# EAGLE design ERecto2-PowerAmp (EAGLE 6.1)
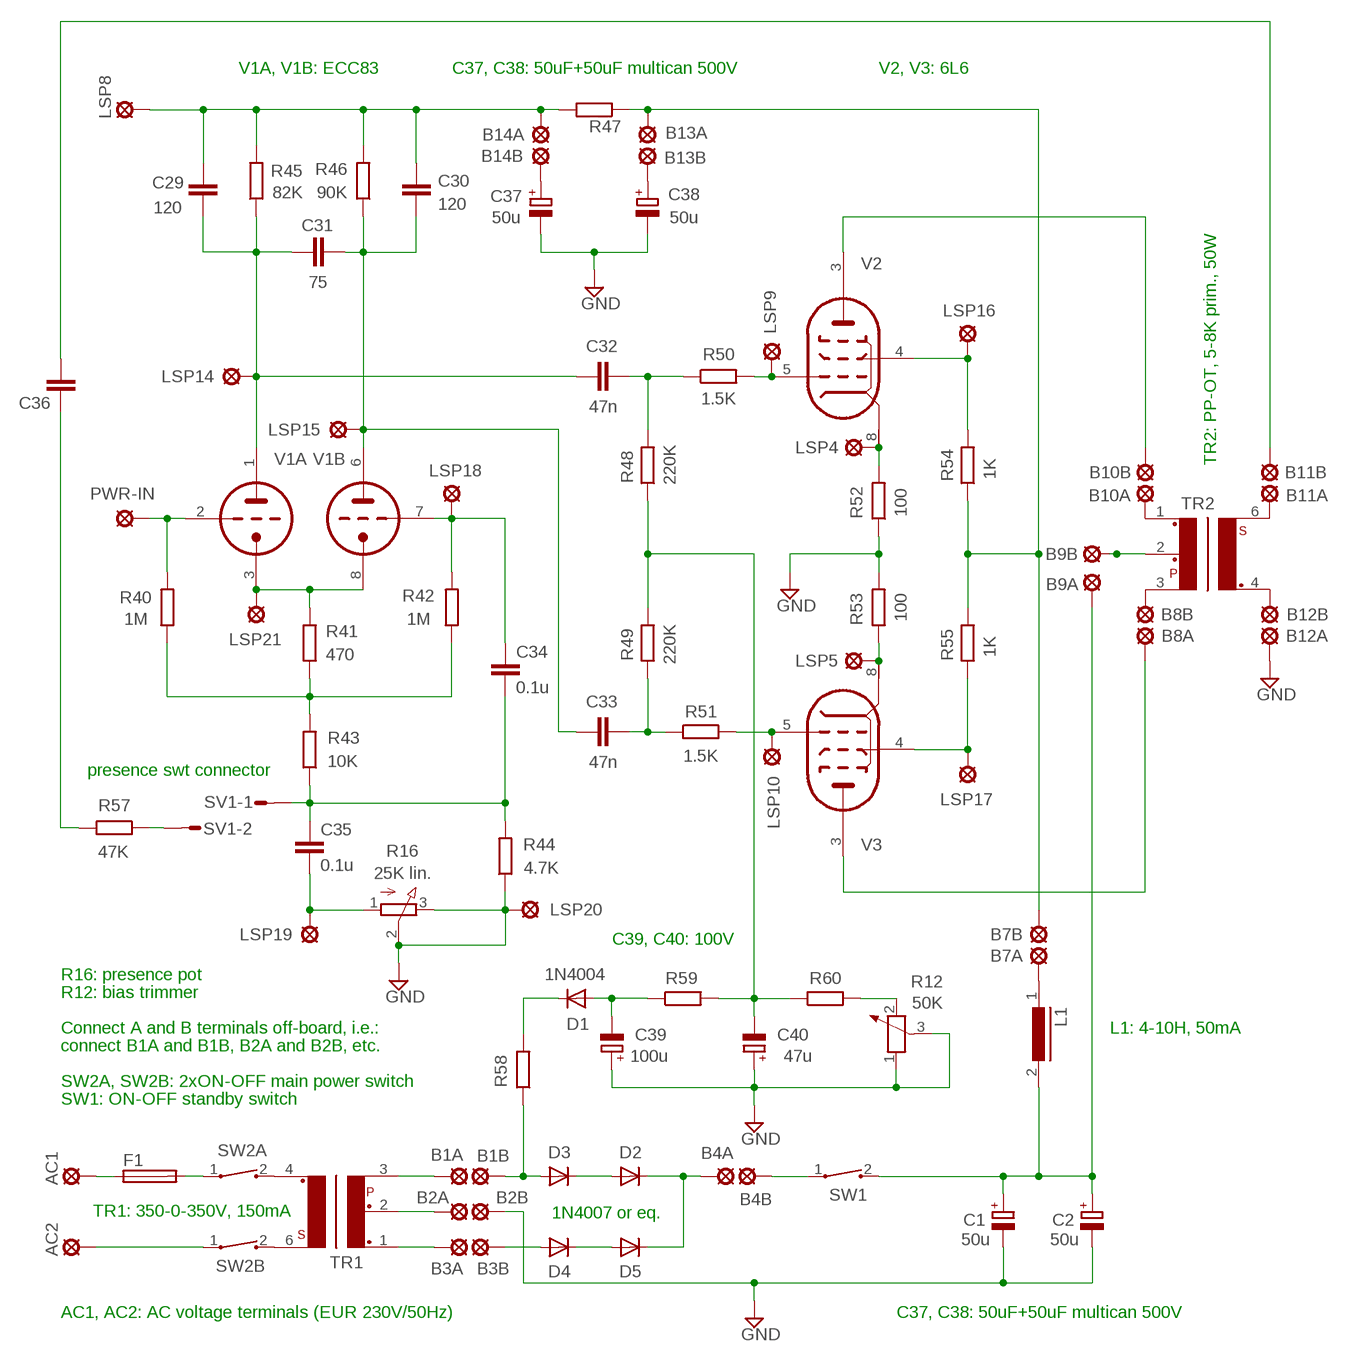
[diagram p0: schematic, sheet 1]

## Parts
AC1  LSP13  [LSP13]
AC2  LSP13  [LSP13]
B1A  LSP13  [LSP13]
B1B  LSP13  [LSP13]
B2A  LSP13  [LSP13]
B2B  LSP13  [LSP13]
B3A  LSP13  [LSP13]
B3B  LSP13  [LSP13]
B4A  LSP13  [LSP13]
B4B  LSP13  [LSP13]
B7A  LSP13  [LSP13]
B7B  LSP13  [LSP13]
B8A  LSP13  [LSP13]
B8B  LSP13  [LSP13]
B9A  LSP13  [LSP13]
B9B  LSP13  [LSP13]
B10A  LSP13  [LSP13]
B10B  LSP13  [LSP13]
B11A  LSP13  [LSP13]
B11B  LSP13  [LSP13]
B12A  LSP13  [LSP13]
B12B  LSP13  [LSP13]
B13A  LSP13  [LSP13]
B13B  LSP13  [LSP13]
B14A  LSP13  [LSP13]
B14B  LSP13  [LSP13]
C1  50u  CPOL-EUE10-35  [EB35D]
C2  50u  CPOL-EUE10-35  [EB35D]
C29  120  C-EU102-054X133  [C102-054X133]
C30  120  C-EU102-054X133  [C102-054X133]
C31  75  C-EU102-054X133  [C102-054X133]
C32  47n  C22/7  [C22.5B7]
C33  47n  C22/7  [C22.5B7]
C34  0.1u  C-EU102-054X133  [C102-054X133]
C35  0.1u  C-EU102-054X133  [C102-054X133]
C36  C-EU102-054X133  [C102-054X133]
C37  50u  CPOL-EUE5-8.5  [E5-8,5]
C38  50u  CPOL-EUE5-8.5  [E5-8,5]
C39  100u  CPOL-EUE5-8.5  [E5-8,5]
C40  47u  CPOL-EUE5-8.5  [E5-8,5]
D1  1N4004  [DO41-10]
D2  1N4004  [DO41-10]
D3  1N4004  [DO41-10]
D4  1N4004  [DO41-10]
D5  1N4004  [DO41-10]
F1  FUSEF456  [F456]
L1  82114A  [82114A]
LSP4  LSP13  [LSP13]
LSP5  LSP13  [LSP13]
LSP8  LSP13  [LSP13]
LSP9  LSP13  [LSP13]
LSP10  LSP13  [LSP13]
LSP14  LSP13  [LSP13]
LSP15  LSP13  [LSP13]
LSP16  LSP13  [LSP13]
LSP17  LSP13  [LSP13]
LSP18  LSP13  [LSP13]
LSP19  LSP13  [LSP13]
LSP20  LSP13  [LSP13]
LSP21  LSP13  [LSP13]
PWR-IN  LSP13  [LSP13]
R12  50K  POTENTIOMETER_PT-10  [PT-10]
R16  25K lin.  3RP/1610N  [3RP/1610N]
R40  1M  R-EU_0207/12  [0207/12]
R41  470  R-EU_0207/10  [0207/10]
R42  1M  R-EU_0207/12  [0207/12]
R43  10K  R-EU_0207/12  [0207/12]
R44  4.7K  R-EU_0207/10  [0207/10]
R45  82K  R-EU_0411/15  [0411/15]
R46  90K  R-EU_0411/15  [0411/15]
R47  R-EU_0617/22  [0617/22]
R48  220K  R-EU_0207/12  [0207/12]
R49  220K  R-EU_0207/12  [0207/12]
R50  1.5K  R-EU_0207/12  [0207/12]
R51  1.5K  R-EU_0207/12  [0207/12]
R52  100  R-EU_0617/17  [0617/17]
R53  100  R-EU_0617/17  [0617/17]
R54  1K  R-EU_0617/22  [0617/22]
R55  1K  R-EU_0617/22  [0617/22]
R57  47K  R-EU_0207/10  [0207/10]
R58  R-EU_0207/12  [0207/12]
R59  R-EU_0207/12  [0207/12]
R60  R-EU_0207/12  [0207/12]
SV1  S02P  [S02P]
SW1  CT10-XXXX-A2  [CT10-XXXX-A2]
SW2A  CT10-XXXX-A2  [CT10-XXXX-A2]
SW2B  CT10-XXXX-A2  [CT10-XXXX-A2]
TR1  42TM113  [42TM]
TR2  42TM113  [42TM]
V1  ECC83-P  [NOVAL]
V2  6L6GC-P  [OKTAL]
V3  6L6GC-P  [OKTAL]

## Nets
GND: B2B.MP B12A.MP C1.- C2.- C37.- C38.- C39.+ C40.+ LSP20.MP R12.1 R12.3 R16.2(S) R16.3(E) R44.1 R52.1 R53.2
N$1: LSP4.MP R52.2 V2.8(PK)
N$2: B4A.MP D2.C D5.C
N$3: LSP5.MP R53.1 V3.8(PK)
N$4: LSP17.MP R55.1 V3.4(PSG)
N$5: LSP16.MP R54.2 V2.4(PSG)
N$6: B14A.MP C29.2 C30.1 LSP8.MP R45.2 R46.2 R47.2
N$7: LSP10.MP R51.2 V3.5(PG)
N$8: LSP9.MP R50.2 V2.5(PG)
N$9: C32.2 R48.2 R50.1
N$10: B10B.MP V2.3(PA)
N$11: C33.2 R49.1 R51.1
N$12: C40.- R48.1 R49.2 R59.2 R60.1
N$13: C39.- D1.A R59.1
N$14: D1.C R58.2
N$15: R12.2 R60.2
N$16: B8A.MP V3.3(PA)
N$17: B7B.MP B13A.MP R47.1 R54.1 R55.2
N$18: D2.A D3.C
N$19: D4.C D5.A
N$20: B1B.MP D3.A R58.1
N$21: B3B.MP D4.A
N$22: C30.2 C31.2 C33.1 LSP15.MP R46.1 V1.6(B:TA)
N$23: C29.1 C31.1 C32.1 LSP14.MP R45.1 V1.1(A:TA)
N$24: LSP21.MP R41.2 V1.3(A:TK) V1.8(B:TK)
N$25: C34.1 LSP18.MP R42.2 V1.7(B:TG)
N$26: R40.1 R41.1 R42.1 R43.2
N$27: C35.2 LSP19.MP R16.1(A)
N$28: C34.2 C35.1 R43.1 R44.2 SV1.1
N$29: R57.1 SV1.2
N$30: C36.1 R57.2
N$31: B11B.MP C36.2
N$32: B9A.MP C1.+ C2.+ L1.2 SW1.2
N$33: B1A.MP TR1.3
N$34: B2A.MP TR1.2
N$35: F1.2 SW2A.1
N$36: AC1.MP F1.1
N$37: AC2.MP SW2B.1
N$38: B3A.MP TR1.1
N$39: PWR-IN.MP R40.2 V1.2(A:TG)
N$40: SW2A.2 TR1.4
N$41: SW2B.2 TR1.6
N$42: B4B.MP SW1.1
N$44: B8B.MP TR2.3
N$45: B9B.MP TR2.2
N$46: B10A.MP TR2.1
N$47: B11A.MP TR2.6
N$48: B12B.MP TR2.4
N$49: B7A.MP L1.1
N$51: B13B.MP C38.+
N$52: B14B.MP C37.+
Unconnected: V1.4(":H1) V1.5(":H3) V1.9(":H2) V2.2(H1) V2.7(H2) V3.2(H1) V3.7(H2)

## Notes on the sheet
- V1A, V1B: ECC83 | C37, C38: 50uF+50uF multican 500V | V2, V3: 6L6
- TR2: PP-OT, 5-8K prim., 50W
- presence swt connector
- C39, C40: 100V
- R16: presence pot
- R12: bias trimmer
- Connect A and B terminals off-board, i.e.: | L1: 4-10H, 50mA
- connect B1A and B1B, B2A and B2B, etc.
- SW2A, SW2B: 2xON-OFF main power switch
- SW1: ON-OFF standby switch
- TR1: 350-0-350V, 150mA | 1N4007 or eq.
- AC1, AC2: AC voltage terminals (EUR 230V/50Hz) | C37, C38: 50uF+50uF multican 500V

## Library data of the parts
AC1 AC2 B1A B1B B2A B2B B3A B3B B4A B4B B7A B7B B8A B8B B9A B9B B10A B10B B11A B11B B12A B12B B13A B13B B14A B14B LSP4 LSP5 LSP8-LSP10 LSP14-LSP21 PWR-IN = solpad:LSP13: SOLDER PAD
C1 C2 C37-C40 = rcl:CPOL-EU: POLARIZED CAPACITOR, European symbol
C29-C31 C34-C36 = rcl:C-EU: CAPACITOR, European symbol
C32 C33 = capacitor-wima:C: CAPACITOR
D1-D5 = diode:1N4004: DIODE
F1 = fuse:FUSE: Fuse; OC_FARNELL: unknown; OC_NEWARK: unknown
L1 = inductors:82114A: INDUCTOR
R12 = rcl:POTENTIOMETER_: Potentiometer
R16 = pot:3RP/1610N: 16mm Potentiometer one level Source: http://www.alphapotentiometers.net/html/16mm_pot_2.html
R40-R55 R57-R60 = rcl:R-EU_: RESISTOR, European symbol
SV1 = con-amp-mt:S02P: AMP MT CONNECTOR; OC_FARNELL: unknown; OC_NEWARK: unknown
SW1 SW2A SW2B = switch-coto:CT10-XXXX-: CT10 Series Molded Switch
TR1 TR2 = trafo-xicon:42TM113: Transformer Mouser 42TLM Series Source: http://www.mouser.com/catalog/specsheets/164267.pdf; OC_FARNELL: unknown; OC_NEWARK: unknown
V1 = tubes:ECC83-P
V2 V3 = tubes:6L6GC-P

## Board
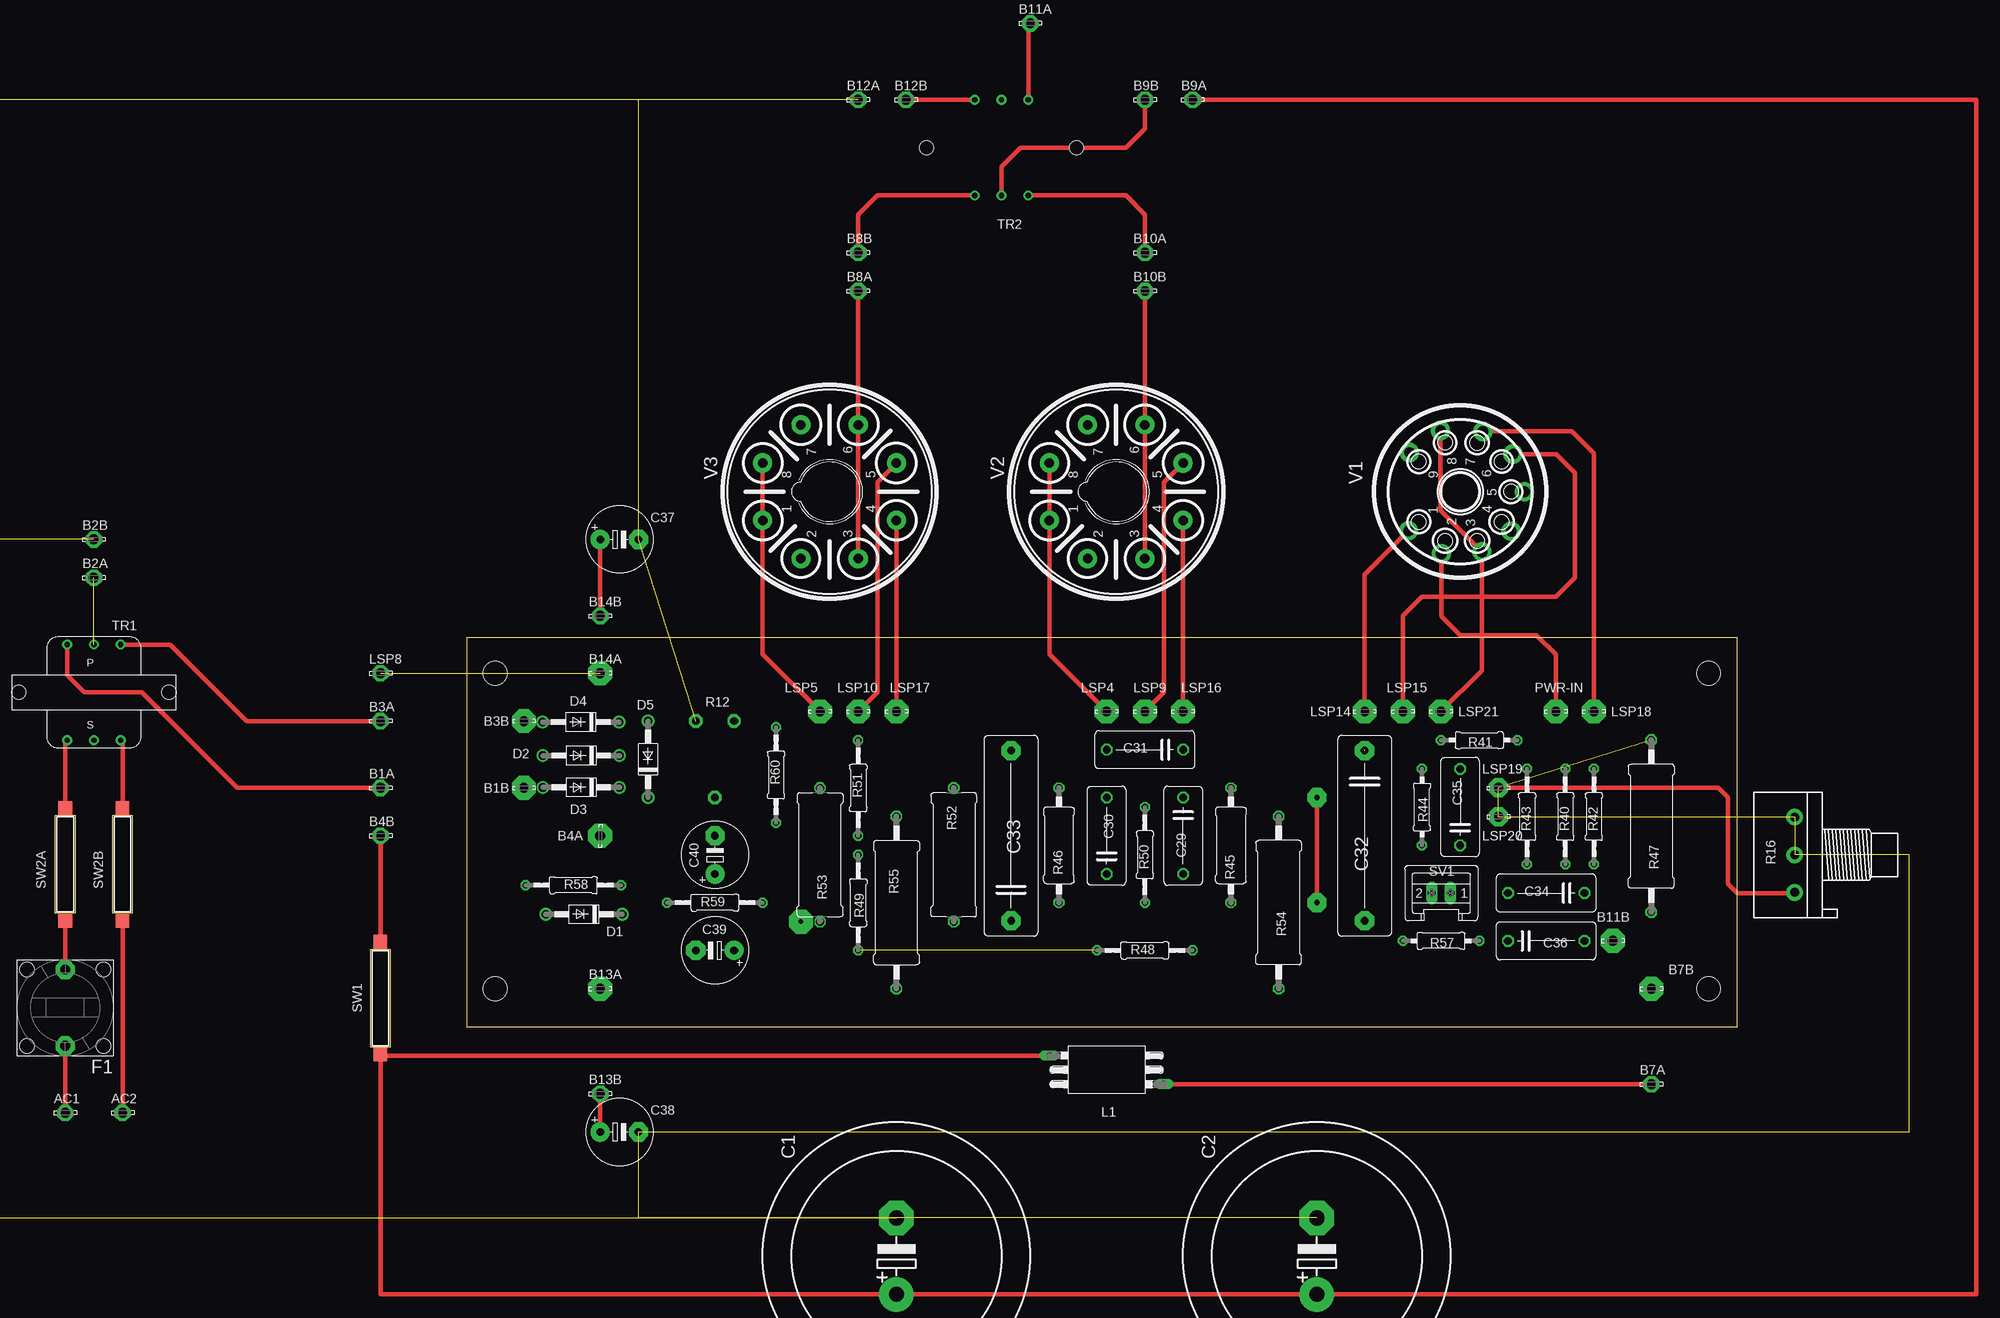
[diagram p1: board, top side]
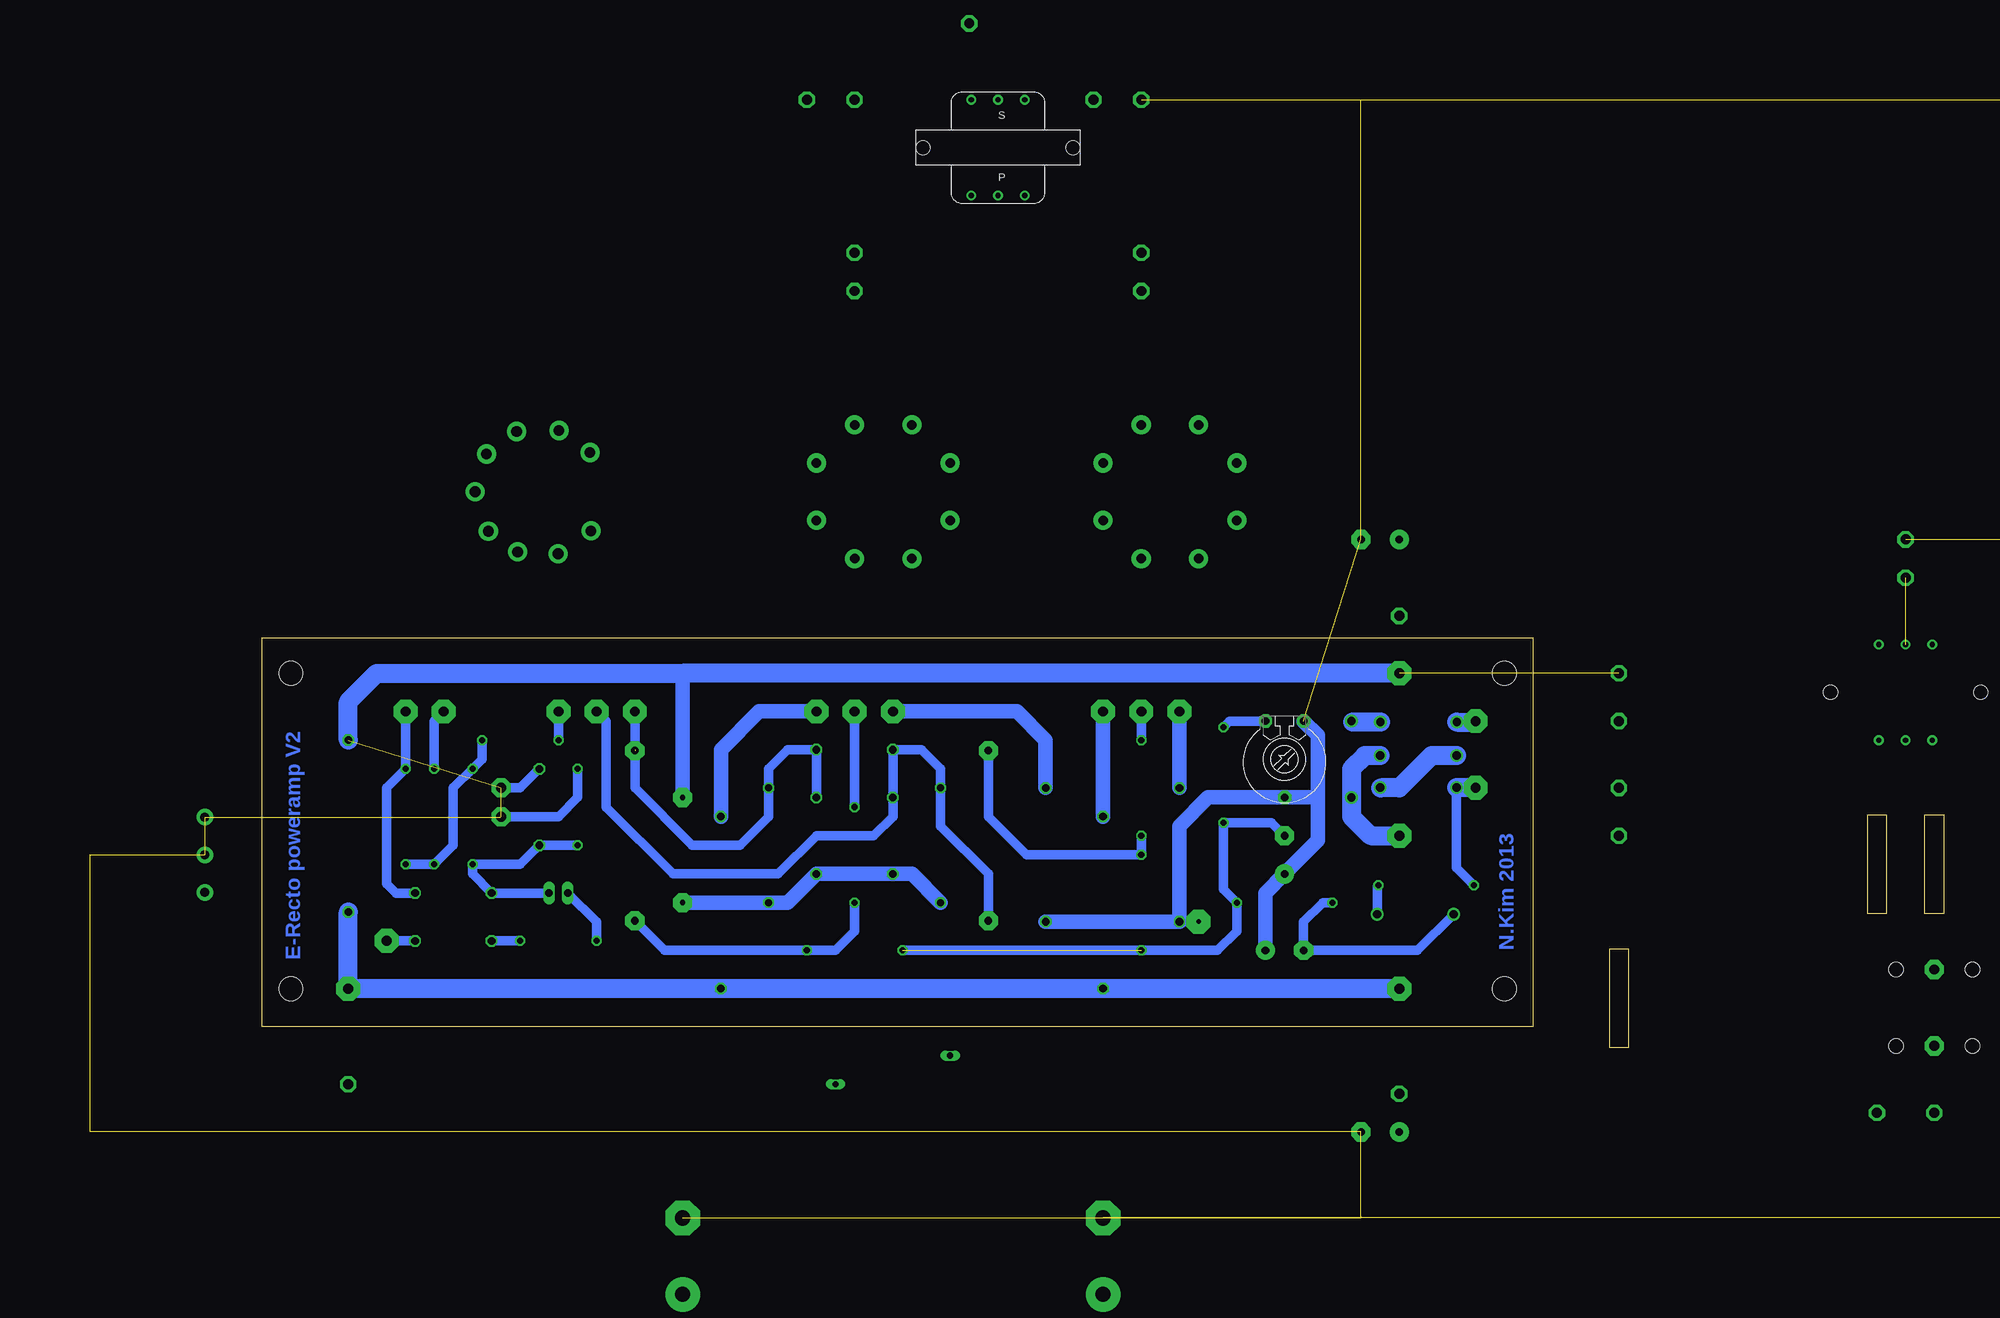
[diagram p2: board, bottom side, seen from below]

Size 223.53 x 54.43 mm. Coordinates in mm from the lower left corner, seen from the top.
Outline: 54.64,2.69 223.53,2.69 223.53,54.43 54.64,54.43 54.64,2.69
Copper layers (1*16): Top 0.035mm / dielectric 1.5mm / Bottom 0.035mm
Design rules: minimum track width 10mil, minimum drill 24mil, track to track 8mil, track to pad 8mil, pad to pad 8mil, via to via 8mil, smd to smd 8mil, copper to edge 40mil, drill to drill 8mil, minimum pad ring 10mil, minimum via ring 8mil, stop-mask expansion 4mil, vias tented up to drill 0mil, thermal gap 10mil
Holes 3.2 mm at 219.74,49.68 219.74,7.77 58.45,49.68 58.45,7.77

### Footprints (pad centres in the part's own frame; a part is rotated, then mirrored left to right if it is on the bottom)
LSP13 = drill 1.321 pad 2.159 octagon: MP 0,0
EB35D = drill 2.007 pad 4.597: + -5.08,0 | drill 2.007 pad 4.597 octagon: - 5.08,0
C102-054X133 = drill 1.016 octagon: 1 -5.08,0; 2 5.08,0
C22.5B7 = drill 1.016 pad 2.54 octagon: 1 -11.303,0; 2 11.303,0
E5-8,5 = drill 1.016 pad 2.54: + -2.54,0 | drill 1.016 pad 2.54 octagon: - 2.54,0
DO41-10 = drill 1.118: A 5.08,0; C -5.08,0
F456 = drill 1.321 pad 2.54 octagon: 1 0,5.08; 2 0,-5.08 | hole 2.007: 5.08,5.08; 5.08,-5.08; -5.08,-5.08; -5.08,5.08
82114A = drill 0.813 long: 1 -7.62,1.905; 2 7.62,-1.905
PT-10 = drill 1.016 pad 1.778 octagon: 1 -2.54,-5.08; 2 2.54,-5.08; 3 0,5.08
3RP/1610N = drill 1.2 pad 2.184: 1 -5,0; 2 0,0; 3 5,0
0207/12 = drill 0.813 octagon: 1 -6.35,0; 2 6.35,0
0207/10 = drill 0.813 octagon: 1 -5.08,0; 2 5.08,0
0411/15 = drill 0.914 octagon: 1 -7.62,0; 2 7.62,0
0617/22 = drill 1.016 octagon: 1 -11.43,0; 2 11.43,0
0617/17 = drill 1.016 octagon: 1 -8.89,0; 2 8.89,0
S02P = drill 1.016 long: 1 1.25,0; 2 -1.25,0
CT10-XXXX-A2 = smd 1.8 x 1.8: 1 -7.5,0; 2 7.5,0
42TM = drill 0.7 pad 1.3: 1 -3.556,-6.35; 2 0,-6.35; 3 3.556,-6.35; 4 3.556,6.35; 5 0,6.35; 6 -3.556,6.35 | hole 1.9: -9.982,0; 9.982,0
NOVAL = drill 1.422 pad 2.54: 1 5.207,-6.858; 2 8.254,-2.484; 3 8.004,2.893; 4 5.258,6.77; 5 0,8.524; 6 -5.004,7.024; 7 -8.004,3.02; 8 -8.127,-2.611; 9 -5.207,-6.731
OKTAL = drill 1.27 pad 2.54: 1 3.81,-8.89; 2 8.89,-3.81; 3 8.89,3.81; 4 3.81,8.89; 5 -3.81,8.89; 6 -8.89,3.81; 7 -8.89,-3.81; 8 -3.81,-8.89

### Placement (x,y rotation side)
AC1  1.3,-8.74 0 top  (outside the outline)
AC2  8.92,-8.74 0 top  (outside the outline)
B1A  43.21,34.44 0 top
B1B  62.26,34.44 0 top
B2A  not placed on the board
B2B  not placed on the board
B3A  43.21,43.33 0 top
B3B  62.26,43.33 0 top
B4A  72.42,28.09 90 top
B4B  43.21,28.09 0 top
B7A  212.12,-4.93 0 top  (outside the outline)
B7B  212.12,7.77 0 top
B8A  106.71,100.48 0 top  (outside the outline)
B8B  106.71,105.56 0 top  (outside the outline)
B9A  151.16,125.88 0 top  (outside the outline)
B9B  144.81,125.88 0 top  (outside the outline)
B10A  144.81,105.56 0 top  (outside the outline)
B10B  144.81,100.48 0 top  (outside the outline)
B11A  129.57,136.04 0 top  (outside the outline)
B11B  207.04,14.12 0 top
B12A  not placed on the board
B12B  113.06,125.88 0 top  (outside the outline)
B13A  72.42,7.77 0 top
B13B  72.42,-6.2 0 top  (outside the outline)
B14A  72.42,49.68 0 top
B14B  72.42,57.3 0 top
C1  111.79,-27.79 90 top  (outside the outline)
C2  167.67,-27.79 90 top  (outside the outline)
C29  149.89,28.09 270 top
C30  139.73,28.09 90 top
C31  144.81,39.52 180 top
C32  174.02,28.09 270 top
C33  127.03,28.09 90 top
C34  198.15,20.47 180 top
C35  186.72,31.9 90 top
C36  198.15,14.12 0 top
C37  74.96,67.46 0 top  (outside the outline)
C38  74.96,-11.28 0 top  (outside the outline)
C39  87.66,12.85 180 top
C40  87.66,25.55 90 top
D1  70.26,17.66 180 top
D2  69.88,38.75 180 top
D3  69.88,34.52 180 top
D4  69.84,43.2 180 top
D5  78.77,38.25 90 top
F1  1.3,5.23 180 top
L1  139.73,-3.02 180 top
LSP4  139.73,44.6 0 top
LSP5  101.63,44.6 0 top
LSP8  43.21,49.68 0 top
LSP9  144.81,44.6 0 top
LSP10  106.71,44.6 0 top
LSP14  174.02,44.6 0 top
LSP15  179.1,44.6 0 top
LSP16  149.89,44.6 0 top
LSP17  111.79,44.6 0 top
LSP18  204.5,44.6 0 top
LSP19  191.8,34.44 0 top
LSP20  191.8,30.63 0 top
LSP21  184.18,44.6 0 top
PWR-IN  199.42,44.6 0 top
R12  87.66,38.25 180 bottom
R16  231.17,25.55 90 top  (outside the outline)
R40  200.69,30.63 90 top
R41  189.26,40.79 180 top
R42  204.5,30.63 90 top
R43  195.61,30.63 90 top
R44  181.64,31.9 270 top
R45  156.24,26.82 270 top
R46  133.38,26.82 270 top
R47  212.12,29.36 90 top
R48  144.81,12.85 0 top
R49  106.71,19.2 270 top
R50  144.81,25.55 90 top
R51  106.71,34.44 90 top
R52  119.41,25.55 90 top
R53  101.63,25.55 270 top
R54  162.59,19.2 90 top
R55  111.79,19.2 270 top
R57  184.18,14.12 0 top
R58  68.85,21.52 0 top
R59  87.66,19.2 0 top
R60  95.78,36.17 90 top
SV1  184.18,20.47 0 top
SW1  43.21,6.5 270 top
SW2A  1.3,24.28 90 top
SW2B  8.92,24.28 90 top
TR1  5.11,47.14 180 top
TR2  125.76,119.53 0 bottom  (outside the outline)
V1  186.72,73.81 270 top  (outside the outline)
V2  141,73.81 270 top  (outside the outline)
V3  102.9,73.81 270 top  (outside the outline)

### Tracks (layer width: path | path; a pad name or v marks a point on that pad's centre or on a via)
GND  (via drill 0.6 pad 3.17)  (16 unrouted)
  Top 0.61: 191.88,30.55 LSP20.MP
  Bottom 1.27: LSP20.MP 184.18,30.63 181.64,33.17 R44.1 | R53.2 v99.09,16.66
  Bottom 1.93: R52.1 R53.2 101.63,29.36 97.82,33.17 R12.3 83.22,33.17 | C39.+ 90.2,20.47 C40.+ 83.22,27.46 83.22,33.17 | 83.22,33.17 83.22,41.43 R12.1
  other vias: 62.26,43.33 62.26,34.44 72.42,49.68 72.42,7.77 101.63,44.6 106.71,44.6 111.79,44.6 174.02,44.6 179.1,44.6 184.18,44.6 139.73,44.6 144.81,44.6 149.89,44.6 199.42,44.6 204.5,44.6 212.12,7.77 207.04,14.12 72.42,28.09
N$1
  Top 0.61: V2.8 132.11,52.22 LSP4.MP
  Bottom 1.93: R52.2 119.41,40.79 123.22,44.6 LSP4.MP
N$2
  Bottom 2.54: D2.C 77,38.75 78.77,36.98 D5.C 78.77,30.63 76.23,28.09 B4A.MP
N$3
  Top 0.61: V3.8 94.01,52.22 LSP5.MP
  Bottom 1.93: R53.1 LSP5.MP
N$4
  Top 0.61: V3.4 LSP17.MP
  Bottom 1.93: LSP17.MP R55.1
N$5
  Top 0.61: V2.4 LSP16.MP
  Bottom 1.93: R54.2 162.59,39.52 157.51,44.6 LSP16.MP
N$6  (via drill 0.7 pad 2.54)  (3 unrouted)
  Top 0.61: v167.67,19.2 v167.67,33.17
  Bottom 1.93: v167.67,33.17 167.67,49.68 | v167.67,19.2 R45.2 153.7,19.2 C29.2 C30.1 137.19,23.01 R46.2
  Bottom 2.54: R47.2 212.12,45.87 208.31,49.68 167.67,49.68 B14A.MP
  other vias: 191.8,34.44 191.8,30.63
N$7
  Top 0.61: V3.5 109.25,75.08 109.25,47.14 LSP10.MP
  Bottom 1.27: R51.2 LSP10.MP
N$8
  Top 0.61: V2.5 147.35,75.08 147.35,47.14 LSP9.MP
  Bottom 1.27: R50.2 LSP9.MP
N$9
  Bottom 1.27: R50.1 144.81,15.39 147.35,12.85 R48.2 170.08,12.85 C32.2
N$10
  Top 0.61: V2.3 B10B.MP
N$11
  Bottom 1.27: R51.1 R49.1 121.95,25.55 127.03,30.63 C33.2
N$12  (1 unrouted)
  Bottom 1.27: C40.- 89.39,29.82 R60.1 95.78,20.97 R59.2 94.01,15.39 96.55,12.85 R48.1
N$13
  Bottom 1.27: R59.1 82.58,19.2 85.12,16.66 C39.- 69.99,12.85 D1.A
N$14
  Bottom 1.27: D1.C 75.34,21.38 R58.2
N$15
  Bottom 1.27: R12.2 94.97,43.33 R60.2
N$16
  Top 0.61: V3.3 B8A.MP
N$17
  Bottom 2.54: R47.1 B7B.MP R54.1 R55.2 B13A.MP
N$18
  Bottom 1.27: 74.88,34.44 D3.C
  Bottom 2.54: D2.A 68.11,38.75 72.42,34.44 74.88,34.44
N$19
  Bottom 1.27: 78.64,43.2 D5.A
  Bottom 2.54: D4.C 78.64,43.2
N$20
  Bottom 1.27: D3.A 64.8,23.82 R58.1
  Bottom 2.54: D3.A 62.34,34.52 B1B.MP
N$21
  Bottom 2.54: D4.A 62.26,43.2 B3B.MP
N$22
  Top 0.61: V1.6 199.5,78.81 201.96,76.35 201.96,62.38 199.42,59.84 181.64,59.84 179.1,57.3 LSP15.MP
  Bottom 1.27: LSP15.MP 177.83,43.33 177.83,31.9 168.94,23.01 154.97,23.01 149.89,28.09 142.27,28.09 139.73,30.63 C30.2 C31.2 135.92,39.52 133.38,36.98 R46.1 133.38,29.36 127.03,23.01 C33.1
N$23  (1 unrouted)
  Top 0.61: V1.1 174.02,62.76 LSP14.MP
  Bottom 1.27: C29.1 C31.1 153.7,39.52 156.24,36.98 R45.1 156.24,30.63 160.05,26.82 166.4,26.82 174.02,34.44 174.02,39.52 LSP14.MP
N$24
  Top 0.61: LSP21.MP 189.61,50.03 V1.3 184.11,71.31 V1.8
  Bottom 1.27: R41.2 LSP21.MP
N$25
  Top 0.61: V1.7 201.58,81.81 204.5,78.89 LSP18.MP
  Bottom 1.27: C34.1 205.77,20.47 207.04,21.74 207.04,34.44 R42.2 LSP18.MP
N$26
  Bottom 1.27: R41.1 194.34,38.25 R43.2 198.15,34.44 198.15,26.82 R40.1 R42.1
N$27
  Top 0.61: LSP19.MP 221.01,34.44 222.28,33.17 222.28,21.74 223.55,20.47 231.09,20.47 R16.1
  Bottom 1.27: LSP19.MP 189.26,34.44 C35.2
N$28
  Bottom 1.27: R44.2 C35.1 189.26,24.28 R43.1 195.61,23.01 C34.2 SV1.1
N$29
  Bottom 1.27: SV1.2 179.1,16.64 R57.1
N$30
  Bottom 1.27: R57.2 C36.1
N$31
  Bottom 1.27: B11B.MP C36.2
N$32
  Top 0.61: B9A.MP 255.3,125.88 255.3,-32.87 C2.+ C1.+ 43.21,-32.87 SW1.2 43.21,-1.12 L1.2
N$33
  Top 0.61: TR1.3 1.55,49.43 3.84,47.14 11.46,47.14 24.16,34.44 B1A.MP
N$34  (1 unrouted)
N$35
  Top 0.61: F1.2 SW2A.1
N$36
  Top 0.61: AC1.MP F1.1
N$37
  Top 0.61: AC2.MP SW2B.1
N$38
  Top 0.61: TR1.1 15.27,53.49 25.43,43.33 B3A.MP
N$39
  Top 0.61: V1.2 184.24,57.24 186.72,54.76 196.88,54.76 199.42,52.22 PWR-IN.MP
  Bottom 1.27: R40.2 200.69,43.33 PWR-IN.MP
N$40
  Top 0.61: SW2A.2 1.3,40.54 TR1.4
N$41
  Top 0.61: SW2B.2 8.92,40.54 TR1.6
N$42
  Top 0.61: SW1.1 B4B.MP
N$44
  Top 0.61: TR2.3 109.25,113.18 106.71,110.64 B8B.MP
N$45
  Top 0.61: TR2.2 125.76,116.99 128.3,119.53 142.27,119.53 144.81,122.07 B9B.MP
N$46
  Top 0.61: TR2.1 142.27,113.18 144.81,110.64 B10A.MP
N$47
  Top 0.61: TR2.6 129.32,136.04 B11A.MP
N$48
  Top 0.61: TR2.4 B12B.MP
N$49
  Top 0.61: L1.1 B7A.MP
N$51
  Top 0.61: C38.+ B13B.MP
N$52
  Top 0.61: B14B.MP C37.+

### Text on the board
Bottom: N.Kim 2013 | E-Recto poweramp V2
Unrouted: GND | GND | GND | GND | GND | GND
